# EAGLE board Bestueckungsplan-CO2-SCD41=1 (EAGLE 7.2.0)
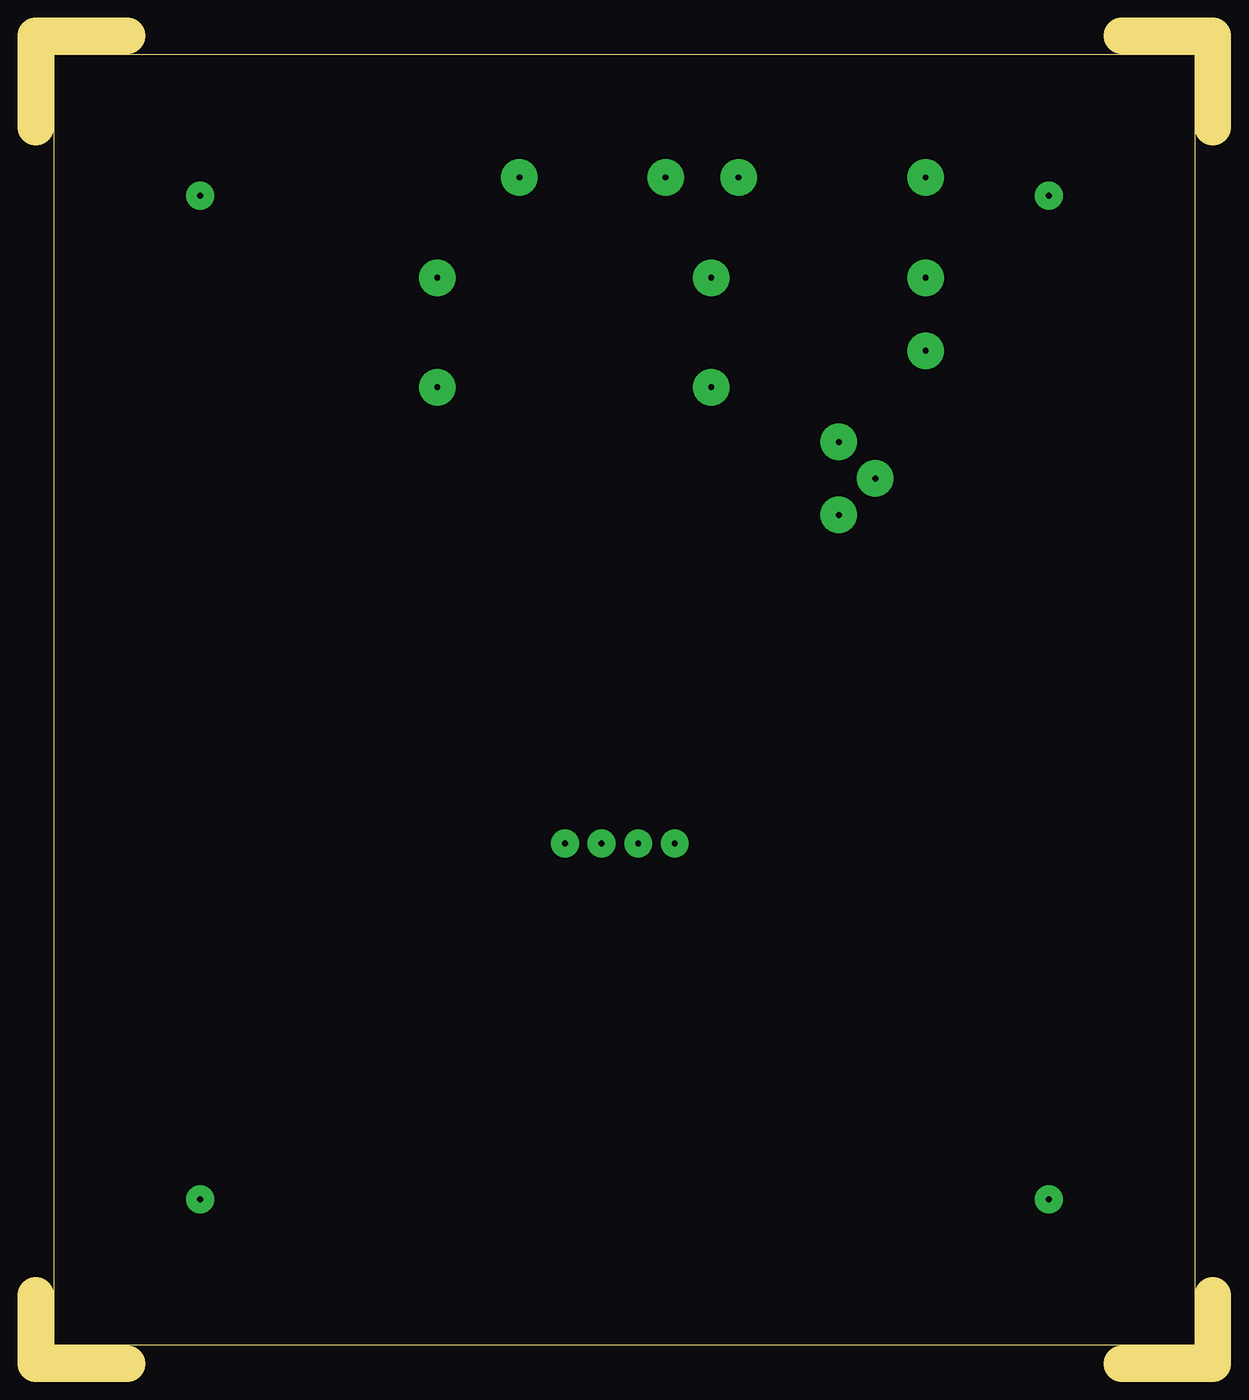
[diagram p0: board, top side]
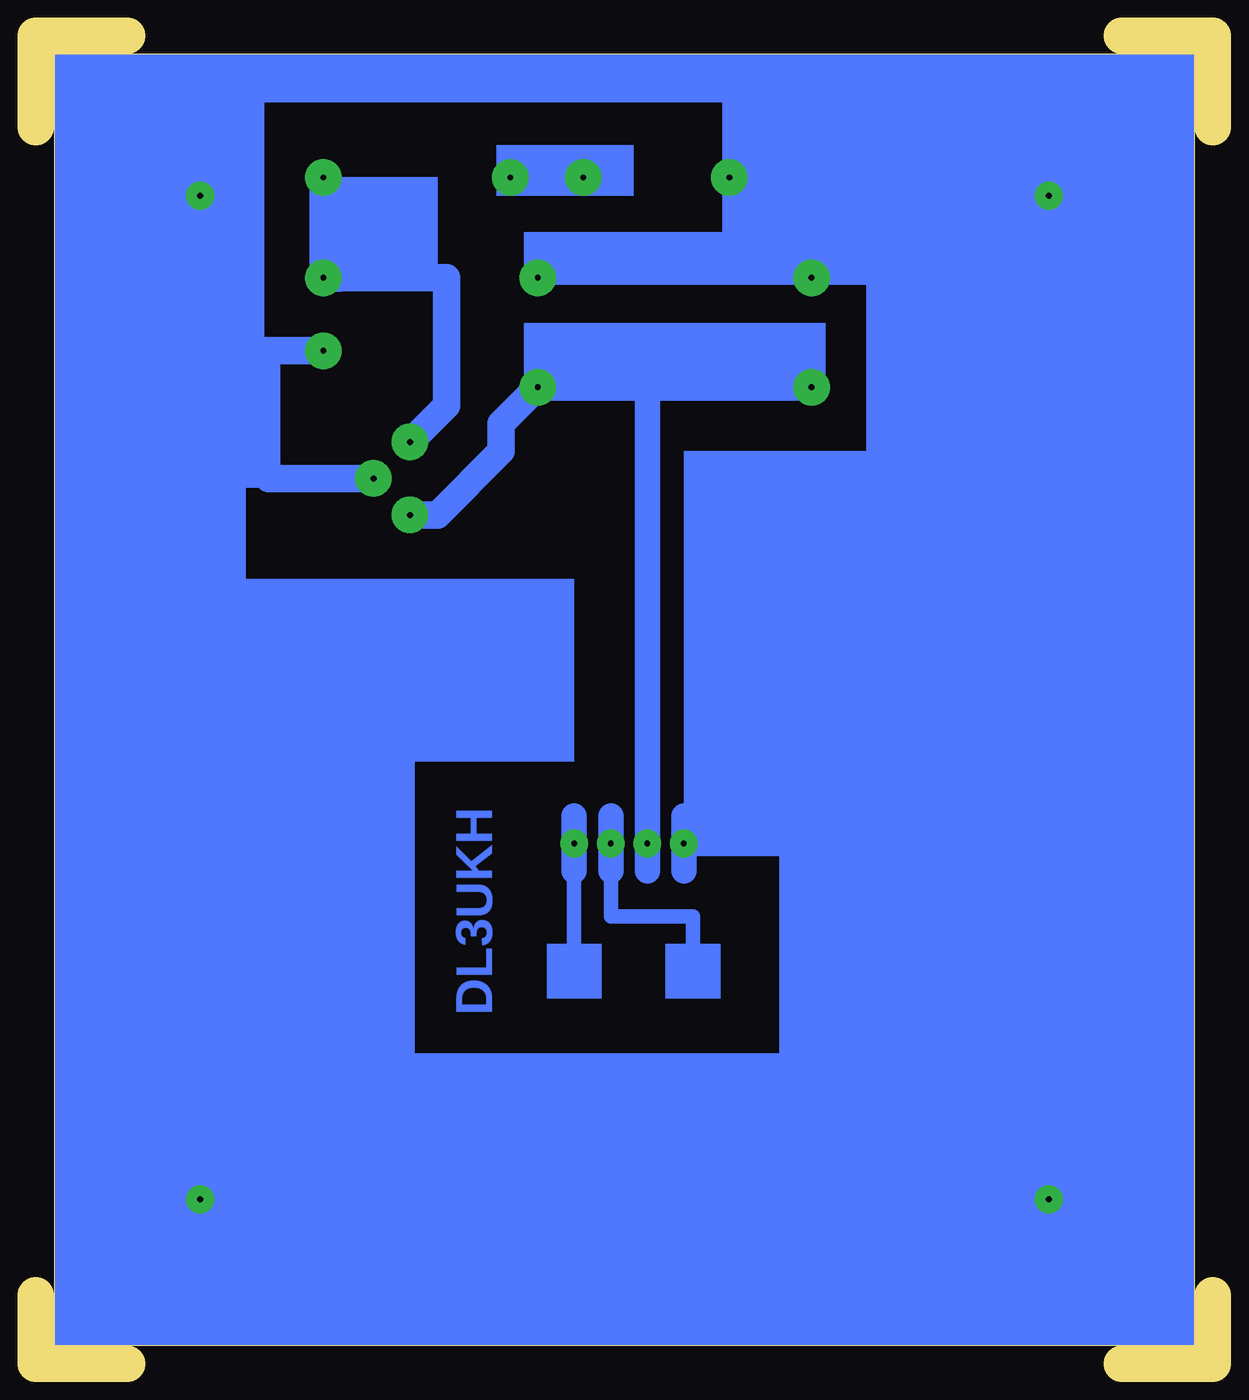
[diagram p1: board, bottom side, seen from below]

Size 81.91 x 92.39 mm. Coordinates in mm from the lower left corner, seen from the top.
Outline: 81.91,86.04 81.91,92.39 75.56,92.39
Outline: 81.91,4.76 81.91,0 75.56,0
Outline: 6.35,0 0,0 0,4.76
Outline: 0,86.04 0,92.39 6.35,92.39
Outline: 80.64,91.12 80.64,1.27 1.27,1.27 1.27,91.12 80.64,91.12
Copper layers (1*16): Top 0.035mm / dielectric 1.5mm / Bottom 0.035mm
Design rules "default": minimum track width 10mil, minimum drill 24mil, track to track 8mil, track to pad 8mil, pad to pad 8mil, via to via 8mil, smd to smd 8mil, copper to edge 40mil, drill to drill 8mil, minimum pad ring 10mil, minimum via ring 8mil, stop-mask expansion 4mil, vias tented up to drill 0mil, thermal gap 10mil

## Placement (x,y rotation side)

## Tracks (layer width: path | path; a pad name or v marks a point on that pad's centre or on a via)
S$1  (via drill 0.4 pad 1.93)
  other vias: 39.37,36.2
S$2  (via drill 0.4 pad 1.93)
  Bottom 1.016: v41.91,36.2 41.91,31.11 36.2,31.11 36.2,27.3
S$3  (via drill 0.4 pad 2.54)
  Bottom 1.93: v43.82,82.55 v48.9,82.55
S$4  (via drill 0.4 pad 1.93)
  Bottom 1.016: v44.45,36.2 44.45,27.3
S$5  (via drill 0.4 pad 2.54)
  Bottom 1.93: v61.91,82.55 v61.91,75.56 53.34,75.56 53.34,66.67 v55.88,64.14
S$6  (via drill 0.4 pad 1.93)
  Bottom 1.016: 20.32,36.2 20.32,33.02 20.32,26.04
  Bottom 1.778: v36.83,36.2 36.83,34.29 | v36.83,36.2 36.83,38.1 | 39.37,34.29 39.37,38.1 39.37,68.9 | 41.91,34.29 41.91,38.1 | 44.45,34.29 44.45,38.1 | v36.83,36.2 20.32,36.2
S$7  (via drill 0.4 pad 2.54)
  Bottom 1.93: v55.88,59.05 53.98,59.05 49.53,63.5 49.53,65.41 v46.99,67.94 v27.94,67.94
S$8  (via drill 0.4 pad 1.93)
  other vias: 11.43,11.43
S$9  (via drill 0.4 pad 1.93)
  other vias: 11.43,81.28
S$10  (via drill 0.4 pad 2.54)
  Bottom 1.016: 20,33.02 12.7,33.02 12.7,75.56 20.32,75.56 | v61.91,70.48 65.41,70.48 | 65.41,70.48 65.41,61.6 58.74,61.6 v58.42,61.6 | 65.41,70.48 66.36,70.48 70.48,70.48 | 70.48,70.48 70.48,88.27 33.66,88.27 v33.66,82.55 33.66,75.56 | 33.66,75.56 v27.94,75.56 20.32,75.56 | 33.66,75.56 v46.99,75.56 | 70.48,70.48 78.42,70.48 78.42,3.17 59.69,3.17 24.77,3.17 | 20.32,33.34 20.32,75.56
  Bottom 1.93: 58.74,61.6 65.72,61.6 | v61.91,70.48 66.36,70.48
S$29  (via drill 0.4 pad 1.93)
  other vias: 70.48,11.43
S$34  (via drill 0.4 pad 1.93)
  other vias: 70.48,81.28
(copper drawn outside any net)
  shapes: Bottom area x34

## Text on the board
Bottom: DL3UKH
Pads: AUF BESTÜCKUNGS-SEITE GESEHEN
Vias: 1 | 2 | 2 | 1 | SCL | SDA
tOrigins: µA7805 | 12 Volt | Kat | - | + | 1N4002 | Eing. | Ausg. | + | Masse | 470µ | 4700µ | 4700µ | - | + | + | Eing. | 1N4002 | 5 Volt | µA7805 | Sensor CO2 | SCD41 | Katode | Anode | Kat | Für Anschlüsse | Siehe Stromlaufplan | Auf Leiterzugseite anlöten | Auch die 5,0Volt | Leiterplatte: | 1,5mm dick | Cevausit | Alles mit 0,8mm vorbohren ! | Aufbohren: | 1N4002 1,0mm | µA7805 1,0mm | 4stck Befestigungs-Bohrungen 3,5mm | 2stck. Elkos 4700µ 1,0mm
